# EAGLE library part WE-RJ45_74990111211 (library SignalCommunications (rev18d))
Order Code 74990111211 Design THT xBase-T 10/100 Base-T Ports 1x1 Application Standard Tab Position UP LED (Left-Right) L-R yellow-green Details see: http://katalog.we-online.de/en/pbs/WE-LAN_RJ45/74990110030?
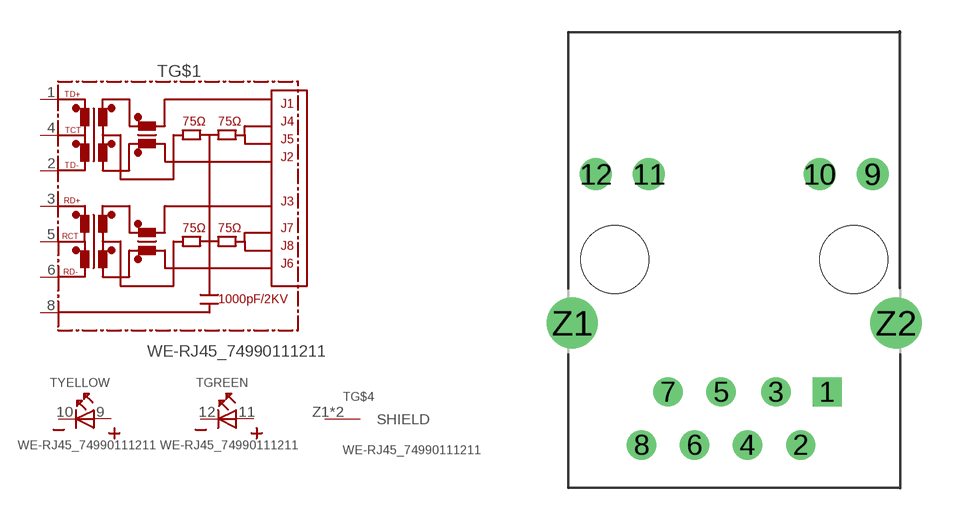
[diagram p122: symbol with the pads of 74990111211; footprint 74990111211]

Designator prefix T; gates G$1=74990111211 YELLOW=LED-2PIN GREEN=LED-2PIN G$4=SHIELD

## WE-RJ45_74990111211  [74990111211]
1  G$1:1
2  G$1:2
3  G$1:3
4  G$1:4
5  G$1:5
6  G$1:6
8  G$1:8
9  YELLOW:A  pas
10  YELLOW:K  pas
11  GREEN:A  pas
12  GREEN:K  pas
Z1  G$4:SHIELD  pas
Z2  G$4:SHIELD  pas

## Footprint 74990111211 (pad centres in mm)
drill 0.89 square: 1 4.45,-6.35
drill 0.89: 2 3.18,-8.89; 3 2,-6.35; 4 0.64,-8.89; 5 -0.63,-6.35; 6 -1.9,-8.89; 7 -3.17,-6.35; 8 -4.44,-8.89
drill 1.02: 9 6.625,4.08; 10 4.085,4.08; 11 -4.085,4.08; 12 -6.625,4.08
drill 1.63: Z1 -7.745,-3.05; Z2 7.745,-3.05
hole 3.25 at -5.715,0
hole 3.25 at 5.715,0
